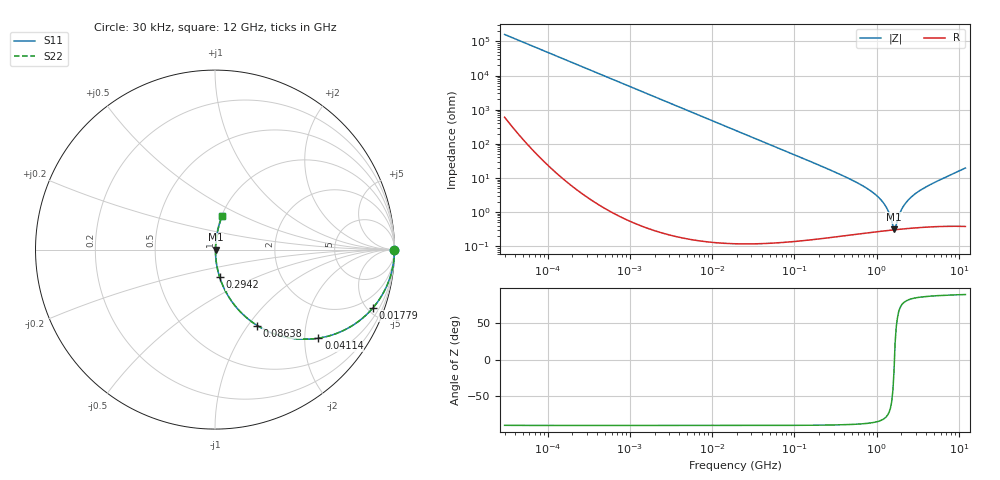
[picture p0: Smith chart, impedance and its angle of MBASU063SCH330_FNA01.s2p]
! MBASU063SCH330_FNA01  S-PARAMETER MODEL  ( General Type )
! Model Generated by TAIYO YUDEN Corporation (http://www.ty-top.com)
! Version 1.0
! TAIYO YUDEN Control No. 130801
! Copyright(c) 2013 TAIYO YUDEN CO.,LTD. All Rights Reserved.
! Product Description (link to TY-COMPAS)
! https://ds.yuden.co.jp/TYCOMPAS/or/detail?pn=MBASU063SCH330JFNA01&u=M
! Products Name : Multilayer Ceramic Capacitors
! Characteristics :
!  Capacitance : 33 pF , Rated Voltage : 50V , TCC : CH / C0H
!  Case Size : 0.6 x 0.3 / 0.024 x 0.012 [mm/inch] , Thickness : 0.3 / 0.012 [mm/inch]
!  (Conditions: Temperature = 25 degC , DC Bias Current/Voltage = 0A / 0V)
! External Node Assignments :
!  1  o---| |---o  2
! GND o---------o GND
! Frequency Range : 0.03MHz  -  12000MHz  [ 401 STEP ]
# MHz S RI R 50
! Freq[MHz].  S11 Real  S11 Imag  S21 Real  S21 Imag  S12 Real  S12 Imag  S22 Real  S22 Imag
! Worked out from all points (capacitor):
!   401 points, 30 kHz to 12 GHz, reference 50 ohm
!   read as one part in series: C = 33.1 pF near 32 kHz
!   lowest |Z| = 316 mohm at 1.625 GHz (marker M1)
!   series resonance near 1.647 GHz, so ESL is about 280 pH
!   S11 on the Smith chart (normalised r, x): 30 kHz: open; 17.79 MHz: 1.00, -5.40; 41.14 MHz: 1.00, -2.33; 86.38 MHz: 1.00, -1.11; 294.2 MHz: 1.00, -0.32; 12 GHz: 1.01, +0.39
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0.03  1 -0.000625  2.73e-06 0.000625  2.73e-06 0.000625  1 -0.000625
0.260295  1 -0.00542  3.04e-05 0.00542  3.04e-05 0.00542  1 -0.00542
2.258455  0.9978 -0.0469  0.00221 0.0469  0.00221 0.0469  0.9978 -0.0469
6.982189  0.9793 -0.1423  0.0207 0.1423  0.0207 0.1423  0.9793 -0.1423
17.78857  0.8793 -0.3256  0.1207 0.3256  0.1207 0.3256  0.8793 -0.3256
18.97367  0.8649 -0.3416  0.1351 0.3416  0.1351 0.3416  0.8649 -0.3416
41.141  0.5765 -0.4936  0.4235 0.4936  0.4235 0.4936  0.5765 -0.4936
86.37604  0.2358 -0.4233  0.7642 0.4233  0.7642 0.4233  0.2358 -0.4233
164.6252  0.0782 -0.2659  0.9218 0.2659  0.9218 0.2659  0.0782 -0.2659
294.1636  0.0261 -0.1537  0.9739 0.1537  0.9739 0.1537  0.0261 -0.1537
579.0248  0.00748 -0.0721  0.9925 0.0721  0.9925 0.0721  0.00748 -0.0721
909.4299  0.00391 -0.0366  0.9961 0.0366  0.9961 0.0366  0.00391 -0.0366
1215.67  0.00312 -0.018  0.9969 0.018  0.9969 0.018  0.00312 -0.018
1428.372  0.00298 -0.00843  0.997 0.00843  0.997 0.00843  0.00298 -0.00843
1573.464  0.00299 -0.00281  0.997 0.00281  0.997 0.00281  0.00299 -0.00281
1625.032  0.00301 -0.000934  0.997 0.000934  0.997 0.000934  0.00301 -0.000934
1733.294  0.00307 0.00307  0.9969 -0.00307  0.9969 -0.00307  0.00307 0.00307
1971.936  0.00326 0.0103  0.9967 -0.0103  0.9967 -0.0103  0.00326 0.0103
2172.242  0.00348 0.0158  0.9965 -0.0158  0.9965 -0.0158  0.00348 0.0158
2903.719  0.00453 0.0331  0.9955 -0.0331  0.9955 -0.0331  0.00453 0.0331
4864.487  0.00857 0.0695  0.9914 -0.0695  0.9914 -0.0695  0.00857 0.0695
12000  0.0404 0.1874  0.9596 -0.1874  0.9596 -0.1874  0.0404 0.1874
